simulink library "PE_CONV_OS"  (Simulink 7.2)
settings: Solver=ode45  SolverMode=SingleTasking  StartTime=0.0  StopTime=10.0  RelTol=1e-3
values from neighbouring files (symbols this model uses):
  C = 10e-3*1    (= 0.01)    [INIT_B6_2L_3Ph_IGBT_OS.m]    (also in INIT_B6_3L_3Ph_IGBT_OS.m; INIT_MMC_100L.m = 0.005; INIT_MMC_200L.m = 0.005; INIT_MMC_20L.m)
  FS = 900    [INIT_B6_2L_3Ph_IGBT_OS.m]    (also in INIT_B6_3L_3Ph_IGBT_OS.m; INIT_PWM_2L.m = 1000; INIT_PWM_3L.m = 1000; INIT_PWM_Con.m = 1000)
  LN = 2e-3    (= 0.002)    [INIT_PWM_2L.m]    (also in INIT_PWM_3L.m; INIT_PWM_Con.m; INIT_MMC_100L.m = 0.025; INIT_MMC_200L.m = 0.025)
  LS = 1e-3    (= 0.001)    [INIT_B6_2L_3Ph_IGBT_OS.m]    (also in INIT_B6_3L_3Ph_IGBT_OS.m; INIT_MMC_100L.m = 0.025; INIT_MMC_200L.m = 0.025; INIT_MMC_20L.m = 0.0025)
  LT = LN    (= 0.025)    [INIT_MMC_100L.m]    (also in INIT_MMC_200L.m; INIT_MMC_20L.m = 0.002; INIT_MMC_400L.m)
  Nc = 100    [INIT_MMC_100L.m]    (also in INIT_MMC_200L.m = 200; INIT_MMC_20L.m = 20; INIT_MMC_400L.m = 400)
  NT = sqrt(3)*340/400    [INIT_MMC_100L.m]    (also in INIT_MMC_200L.m; INIT_MMC_20L.m = sqrt(3); INIT_MMC_400L.m)
  Rg = 1e-3    (= 0.001)    [INIT_MMC_100L.m]    (also in INIT_MMC_200L.m; INIT_MMC_20L.m; INIT_MMC_400L.m)
  RN = 0.1    [INIT_PWM_2L.m]    (also in INIT_PWM_3L.m; INIT_PWM_Con.m; INIT_MMC_100L.m; INIT_MMC_200L.m)
  RT = RN    (= 0.1)    [INIT_MMC_100L.m]    (also in INIT_MMC_200L.m; INIT_MMC_20L.m; INIT_MMC_400L.m)
  UC0 = 600    [INIT_B6_2L_3Ph_IGBT_OS.m]    (also in INIT_B6_3L_3Ph_IGBT_OS.m = 500; INIT_MMC_100L.m = 6800; INIT_MMC_200L.m = 3400; INIT_MMC_20L.m = 5000)
undefined symbols (not defined in the file or in its folder): A, DT, FT, L, O1, O2, PHT, T, Td
libraries: simulink_extras x2
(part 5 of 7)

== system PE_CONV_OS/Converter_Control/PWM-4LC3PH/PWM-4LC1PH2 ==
  In1 : Inport  OutDataType=sfix(16)  OutScaling=2^0
  Mux : Mux  Inputs=6
  PWM-2L-1PH : Subsystem  mask(PWM-2L-1PH){FT=FT, PHT=PHT1, DT=DT}
      mask prompts: FT "Triangular Frequency"; PHT "Trian. Phase Angle (Degree)"; DT "Dead Time"
      mask help: Pulse Width Modulation for 1 Phase Converter
  PWM-2L-1PH1 : Subsystem  mask(PWM-2L-1PH){FT=FT, PHT=PHT2, DT=DT}
      mask prompts: FT "Triangular Frequency"; PHT "Trian. Phase Angle (Degree)"; DT "Dead Time"
      mask help: Pulse Width Modulation for 1 Phase Converter
  PWM-2L-1PH2 : Subsystem  mask(PWM-2L-1PH){FT=FT, PHT=PHT3, DT=DT}
      mask prompts: FT "Triangular Frequency"; PHT "Trian. Phase Angle (Degree)"; DT "Dead Time"
      mask help: Pulse Width Modulation for 1 Phase Converter
  Out1 : Outport
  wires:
  PWM-2L-1PH/2(Out2) -> Mux/6
  In1/1 -> PWM-2L-1PH/1(In1), PWM-2L-1PH1/1(In1), PWM-2L-1PH2/1(In1)
  Mux/1 -> Out1/1
  PWM-2L-1PH2/2(Out2) -> Mux/4
  PWM-2L-1PH2/1(Out1) -> Mux/3
  PWM-2L-1PH1/2(Out2) -> Mux/5
  PWM-2L-1PH1/1(Out1) -> Mux/2
  PWM-2L-1PH/1(Out1) -> Mux/1

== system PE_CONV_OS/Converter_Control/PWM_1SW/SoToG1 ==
  Clock : Clock
  P : Product  OutDataType=sfix(16)  OutScaling=2^0
  T1 : Constant  Value=T  OutDataType=sfix(16)  OutScaling=2^0
  T2 : Constant  Value=1/T  OutDataType=sfix(16)  OutScaling=2^0
  mod : Math  Operator=mod
  O : Outport
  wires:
  P/1 -> O/1
  mod/1 -> P/1
  T2/1 -> P/2
  T1/1 -> mod/2
  Clock/1 -> mod/1

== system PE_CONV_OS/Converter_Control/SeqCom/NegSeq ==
  In1 : Inport  OutDataType=sfix(16)  OutScaling=2^0
  Demux : Demux  Outputs=3
  Gain : Gain  Gain=1/3  ParameterDataType=sfix(16)  ParameterScaling=2^0  OutDataType=sfix(16)  OutScaling=2^0
  Gain1 : Gain  Gain=1/3  ParameterDataType=sfix(16)  ParameterScaling=2^0  OutDataType=sfix(16)  OutScaling=2^0
  Gain2 : Gain  Gain=1/3  ParameterDataType=sfix(16)  ParameterScaling=2^0  OutDataType=sfix(16)  OutScaling=2^0
  Mux : Mux  Inputs=3
  Sum : Sum  Inputs=+++  OutDataType=sfix(16)  OutScaling=2^0
  Sum1 : Sum  Inputs=+++  OutDataType=sfix(16)  OutScaling=2^0
  Sum2 : Sum  Inputs=+++  OutDataType=sfix(16)  OutScaling=2^0
  TD : TransportDelay  DelayTime=T/3  BufferSize=BF
  TD1 : TransportDelay  DelayTime=2*T/3  BufferSize=BF
  TD2 : TransportDelay  DelayTime=2*T/3  BufferSize=BF
  TD3 : TransportDelay  DelayTime=T/3  BufferSize=BF
  TD4 : TransportDelay  DelayTime=T/3  BufferSize=BF
  TD5 : TransportDelay  DelayTime=2*T/3  BufferSize=BF
  Out1 : Outport
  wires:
  Gain2/1 -> Mux/3
  Gain1/1 -> Mux/2
  Sum/1 -> Gain/1
  Demux/1 -> Sum/1, TD2/1, TD4/1
  TD1/1 -> Sum/3
  TD/1 -> Sum/2
  Demux/3 -> TD1/1, TD3/1, Sum2/3
  Demux/2 -> TD/1, Sum1/2, TD5/1
  In1/1 -> Demux/1
  TD2/1 -> Sum1/1
  TD3/1 -> Sum1/3
  Sum1/1 -> Gain1/1
  Gain/1 -> Mux/1
  Mux/1 -> Out1/1
  Sum2/1 -> Gain2/1
  TD4/1 -> Sum2/1
  TD5/1 -> Sum2/2

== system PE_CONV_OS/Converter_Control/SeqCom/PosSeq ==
  In1 : Inport  OutDataType=sfix(16)  OutScaling=2^0
  Demux : Demux  Outputs=3
  Gain : Gain  Gain=1/3  ParameterDataType=sfix(16)  ParameterScaling=2^0  OutDataType=sfix(16)  OutScaling=2^0
  Gain1 : Gain  Gain=1/3  ParameterDataType=sfix(16)  ParameterScaling=2^0  OutDataType=sfix(16)  OutScaling=2^0
  Gain2 : Gain  Gain=1/3  ParameterDataType=sfix(16)  ParameterScaling=2^0  OutDataType=sfix(16)  OutScaling=2^0
  Mux : Mux  Inputs=3
  Sum : Sum  Inputs=+++  OutDataType=sfix(16)  OutScaling=2^0
  Sum1 : Sum  Inputs=+++  OutDataType=sfix(16)  OutScaling=2^0
  Sum2 : Sum  Inputs=+++  OutDataType=sfix(16)  OutScaling=2^0
  TD : TransportDelay  DelayTime=2*T/3  BufferSize=BF
  TD1 : TransportDelay  DelayTime=T/3  BufferSize=BF
  TD2 : TransportDelay  DelayTime=T/3  BufferSize=BF
  TD3 : TransportDelay  DelayTime=2*T/3  BufferSize=BF
  TD4 : TransportDelay  DelayTime=2*T/3  BufferSize=BF
  TD5 : TransportDelay  DelayTime=T/3  BufferSize=BF
  Out1 : Outport
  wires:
  Gain2/1 -> Mux/3
  TD5/1 -> Sum2/2
  TD4/1 -> Sum2/1
  Sum2/1 -> Gain2/1
  Mux/1 -> Out1/1
  Gain1/1 -> Mux/2
  Gain/1 -> Mux/1
  Sum1/1 -> Gain1/1
  TD3/1 -> Sum1/3
  TD2/1 -> Sum1/1
  In1/1 -> Demux/1
  Demux/2 -> TD5/1, Sum1/2, TD/1
  Demux/3 -> Sum2/3, TD3/1, TD1/1
  TD/1 -> Sum/2
  TD1/1 -> Sum/3
  Demux/1 -> TD4/1, TD2/1, Sum/1
  Sum/1 -> Gain/1

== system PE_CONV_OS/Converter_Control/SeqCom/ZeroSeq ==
  In1 : Inport  OutDataType=sfix(16)  OutScaling=2^0
  Demux : Demux  Outputs=3
  Gain : Gain  Gain=1/3  ParameterDataType=sfix(16)  ParameterScaling=2^0  OutDataType=sfix(16)  OutScaling=2^0
  Mux : Mux  Inputs=3
  Sum : Sum  Inputs=+++  OutDataType=sfix(16)  OutScaling=2^0
  Out1 : Outport
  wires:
  Mux/1 -> Out1/1
  Gain/1 -> Mux/3, Mux/1, Mux/2
  In1/1 -> Demux/1
  Sum/1 -> Gain/1
  Demux/1 -> Sum/1
  Demux/2 -> Sum/2
  Demux/3 -> Sum/3

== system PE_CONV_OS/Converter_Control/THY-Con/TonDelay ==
  s1 : Inport  Orientation=down  OutDataType=sfix(16)  OutScaling=2^0
  Int : Integrator  ExternalReset=falling
  Rel1 : Relay  OnSwitchValue=DT  OutDataType=sfix(16)  OutScaling=2^0
  s1d : Outport  InitialOutput=0
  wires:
  Rel1/1 -> s1d/1
  s1/1 -> Int/1, Int/2
  Int/1 -> Rel1/1

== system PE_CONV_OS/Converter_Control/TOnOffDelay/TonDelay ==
  s1 : Inport  Orientation=down  OutDataType=sfix(16)  OutScaling=2^0
  Int : Integrator  ExternalReset=falling
  Rel1 : Relay  OnSwitchValue=DT  OutDataType=sfix(16)  OutScaling=2^0
  s1d : Outport  InitialOutput=0
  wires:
  Rel1/1 -> s1d/1
  s1/1 -> Int/1, Int/2
  Int/1 -> Rel1/1

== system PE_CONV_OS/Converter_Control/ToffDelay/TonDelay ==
  s1 : Inport  Orientation=down  OutDataType=sfix(16)  OutScaling=2^0
  Int : Integrator  ExternalReset=falling
  Rel1 : Relay  OnSwitchValue=DT  OutDataType=sfix(16)  OutScaling=2^0
  s1d : Outport  InitialOutput=0
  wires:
  Int/1 -> Rel1/1
  s1/1 -> Int/2, Int/1
  Rel1/1 -> s1d/1

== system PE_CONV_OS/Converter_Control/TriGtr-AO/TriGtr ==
  Clock : Clock
  S1 : Subsystem
  Sum : Sum
  T : Constant  Value=T
  Td : Constant  Value=Td
  mod : Math  Operator=mod
  O : Outport  InitialOutput=0
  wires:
  mod/1 -> S1/1(I1)
  S1/1(O1) -> O/1
  Clock/1 -> Sum/1
  T/1 -> mod/2
  Sum/1 -> mod/1
  Td/1 -> Sum/2

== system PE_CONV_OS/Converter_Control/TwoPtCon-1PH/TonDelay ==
  s1 : Inport  Orientation=down  OutDataType=sfix(16)  OutScaling=2^0
  Int : Integrator  ExternalReset=falling
  Rel1 : Relay  OnSwitchValue=DT  OutDataType=sfix(16)  OutScaling=2^0
  s1d : Outport  InitialOutput=0
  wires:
  Rel1/1 -> s1d/1
  s1/1 -> Int/1, Int/2
  Int/1 -> Rel1/1

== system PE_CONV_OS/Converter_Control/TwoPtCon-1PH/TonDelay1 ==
  s1 : Inport  Orientation=down  OutDataType=sfix(16)  OutScaling=2^0
  Int : Integrator  ExternalReset=falling
  Rel1 : Relay  OnSwitchValue=DT  OutDataType=sfix(16)  OutScaling=2^0
  s1d : Outport  InitialOutput=0
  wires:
  Rel1/1 -> s1d/1
  s1/1 -> Int/1, Int/2
  Int/1 -> Rel1/1

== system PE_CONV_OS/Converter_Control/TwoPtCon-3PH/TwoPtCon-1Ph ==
  In1 : Inport  OutDataType=sfix(16)  OutScaling=2^0
  In2 : Inport  Port=2  OutDataType=sfix(16)  OutScaling=2^0
  DT : DataTypeConversion
  DT1 : DataTypeConversion
  Relay : Relay  OnSwitchValue=SP  OffSwitchValue=SN  OutDataType=sfix(16)  OutScaling=2^0
  Sum : Sum  Inputs=+-  OutDataType=sfix(16)  OutScaling=2^0
  TonDelay : Subsystem  mask(TonDelay){DT=DT}
      mask prompts: DT "Dead Time"
      mask help: Turn on dead time to protect against short circuit of the converter leg
  TonDelay1 : Subsystem  mask(TonDelay){DT=DT}
      mask prompts: DT "Dead Time"
      mask help: Turn on dead time to protect against short circuit of the converter leg
  not : Logic  Operator=NOT  Inputs=1
  Out1 : Outport  InitialOutput=0
  Out2 : Outport  Port=2  InitialOutput=0
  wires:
  In1/1 -> Sum/1
  In2/1 -> Sum/2
  Sum/1 -> Relay/1
  not/1 -> DT/1
  Relay/1 -> TonDelay/1(s1), DT1/1
  TonDelay1/1(s1d) -> Out2/1
  TonDelay/1(s1d) -> Out1/1
  DT/1 -> TonDelay1/1(s1)
  DT1/1 -> not/1

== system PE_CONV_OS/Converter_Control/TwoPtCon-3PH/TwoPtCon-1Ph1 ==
  In1 : Inport  OutDataType=sfix(16)  OutScaling=2^0
  In2 : Inport  Port=2  OutDataType=sfix(16)  OutScaling=2^0
  DT : DataTypeConversion
  DT1 : DataTypeConversion
  Relay : Relay  OnSwitchValue=SP  OffSwitchValue=SN  OutDataType=sfix(16)  OutScaling=2^0
  Sum : Sum  Inputs=+-  OutDataType=sfix(16)  OutScaling=2^0
  TonDelay : Subsystem  mask(TonDelay){DT=DT}
      mask prompts: DT "Dead Time"
      mask help: Turn on dead time to protect against short circuit of the converter leg
  TonDelay1 : Subsystem  mask(TonDelay){DT=DT}
      mask prompts: DT "Dead Time"
      mask help: Turn on dead time to protect against short circuit of the converter leg
  not : Logic  Operator=NOT  Inputs=1
  Out1 : Outport  InitialOutput=0
  Out2 : Outport  Port=2  InitialOutput=0
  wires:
  In1/1 -> Sum/1
  In2/1 -> Sum/2
  Sum/1 -> Relay/1
  not/1 -> DT/1
  Relay/1 -> TonDelay/1(s1), DT1/1
  TonDelay1/1(s1d) -> Out2/1
  TonDelay/1(s1d) -> Out1/1
  DT/1 -> TonDelay1/1(s1)
  DT1/1 -> not/1

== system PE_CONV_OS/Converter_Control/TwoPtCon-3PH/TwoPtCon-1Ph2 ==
  In1 : Inport  OutDataType=sfix(16)  OutScaling=2^0
  In2 : Inport  Port=2  OutDataType=sfix(16)  OutScaling=2^0
  DT : DataTypeConversion
  DT1 : DataTypeConversion
  Relay : Relay  OnSwitchValue=SP  OffSwitchValue=SN  OutDataType=sfix(16)  OutScaling=2^0
  Sum : Sum  Inputs=+-  OutDataType=sfix(16)  OutScaling=2^0
  TonDelay : Subsystem  mask(TonDelay){DT=DT}
      mask prompts: DT "Dead Time"
      mask help: Turn on dead time to protect against short circuit of the converter leg
  TonDelay1 : Subsystem  mask(TonDelay){DT=DT}
      mask prompts: DT "Dead Time"
      mask help: Turn on dead time to protect against short circuit of the converter leg
  not : Logic  Operator=NOT  Inputs=1
  Out1 : Outport  InitialOutput=0
  Out2 : Outport  Port=2  InitialOutput=0
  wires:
  In1/1 -> Sum/1
  In2/1 -> Sum/2
  Sum/1 -> Relay/1
  not/1 -> DT/1
  Relay/1 -> TonDelay/1(s1), DT1/1
  TonDelay1/1(s1d) -> Out2/1
  TonDelay/1(s1d) -> Out1/1
  DT/1 -> TonDelay1/1(s1)
  DT1/1 -> not/1

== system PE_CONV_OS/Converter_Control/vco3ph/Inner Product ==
  in_1 : Inport  OutDataType=sfix(16)  OutScaling=2^0
  in_2 : Inport  Port=2  OutDataType=sfix(16)  OutScaling=2^0
  Product : Product  OutDataType=sfix(16)  OutScaling=2^0
  Sum : Sum  Inputs=+  OutDataType=sfix(16)  OutScaling=2^0
  out_1 : Outport  InitialOutput=0
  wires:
  Sum/1 -> out_1/1
  Product/1 -> Sum/1
  in_1/1 -> Product/1
  in_2/1 -> Product/2

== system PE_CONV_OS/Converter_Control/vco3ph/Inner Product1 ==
  in_1 : Inport  OutDataType=sfix(16)  OutScaling=2^0
  in_2 : Inport  Port=2  OutDataType=sfix(16)  OutScaling=2^0
  Product : Product  OutDataType=sfix(16)  OutScaling=2^0
  Sum : Sum  Inputs=+  OutDataType=sfix(16)  OutScaling=2^0
  out_1 : Outport  InitialOutput=0
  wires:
  Sum/1 -> out_1/1
  Product/1 -> Sum/1
  in_1/1 -> Product/1
  in_2/1 -> Product/2

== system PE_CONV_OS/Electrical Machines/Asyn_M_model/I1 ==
  Phir* : Inport
  KF : Gain  Gain=1/LM
  Id* : Outport
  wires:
  Phir*/1 -> KF/1
  KF/1 -> Id*/1

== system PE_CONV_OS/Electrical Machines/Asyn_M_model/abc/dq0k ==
  abc : Inport
  th : Inport  Port=2
  Demux : Demux  Outputs=3
  Fcn : Fcn  Expr=u(1)*cos(u(3)) + u(2)*sin(u(3))
  Fcn1 : Fcn  Expr=-u(1)*sin(u(3)) + u(2)*cos(u(3))
  K : Gain  Gain="2/3*[1   -.5   -.5;  0   sqrt(3)/2   -sqrt(3)/2;  .5    .5    .5]"  Multiplication=Matrix(K*u)
  Mux1 : Mux  Inputs=3
  dk : Outport
  qk : Outport  Port=2
  0k : Outport  Port=3
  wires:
  abc/1 -> K/1
  Demux/2 -> Mux1/2
  Demux/1 -> Mux1/1
  Demux/3 -> 0k/1
  th/1 -> Mux1/3
  Fcn1/1 -> qk/1
  Fcn/1 -> dk/1
  Mux1/1 -> Fcn/1, Fcn1/1
  K/1 -> Demux/1

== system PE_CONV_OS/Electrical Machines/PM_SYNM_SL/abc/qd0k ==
  a : Inport  OutDataType=sfix(16)  OutScaling=2^0
  b : Inport  Port=2  OutDataType=sfix(16)  OutScaling=2^0
  c : Inport  Port=3  OutDataType=sfix(16)  OutScaling=2^0
  th : Inport  Port=4  OutDataType=sfix(16)  OutScaling=2^0
  Demux : Demux  Outputs=3
  Fcn : Fcn  Expr=u(1)*cos(u(3)) - u(2)*sin(u(3))
  Fcn1 : Fcn  Expr=u(1)*sin(u(3)) + u(2)*cos(u(3))
  K : Gain  Gain="2/3*[1   -.5   -.5;  0   -sqrt(3)/2   sqrt(3)/2;  .5    .5    .5]"  Multiplication=Matrix(K*u)  ParameterDataType=sfix(16)  ParameterScaling=2^0  OutDataType=sfix(16)  OutScaling=2^0
  Mux : Mux  Inputs=3
  Mux1 : Mux  Inputs=3
  qk : Outport
  dk : Outport  Port=2
  0k : Outport  Port=3
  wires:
  Demux/2 -> Mux1/2
  Demux/1 -> Mux1/1
  Demux/3 -> 0k/1
  th/1 -> Mux1/3
  Fcn1/1 -> dk/1
  Fcn/1 -> qk/1
  Mux1/1 -> Fcn/1, Fcn1/1
  a/1 -> Mux/1
  Mux/1 -> K/1
  K/1 -> Demux/1
  b/1 -> Mux/2
  c/1 -> Mux/3

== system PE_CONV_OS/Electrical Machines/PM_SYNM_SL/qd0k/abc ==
  qk : Inport  OutDataType=sfix(16)  OutScaling=2^0
  dk : Inport  Port=2  OutDataType=sfix(16)  OutScaling=2^0
  0k : Inport  Port=3  OutDataType=sfix(16)  OutScaling=2^0
  th : Inport  Port=4  OutDataType=sfix(16)  OutScaling=2^0
  Demux : Demux  Outputs=3
  Fcn : Fcn  Expr=u(1)*cos(u(3)) + u(2)*sin(u(3))
  Fcn1 : Fcn  Expr=-u(1)*sin(u(3)) + u(2)*cos(u(3))
  K : Gain  Gain="[1   0  1 ;  -.5   -sqrt(3)/2    1 ;  -.5    sqrt(3)/2    1]"  Multiplication=Matrix(K*u)  ParameterDataType=sfix(16)  ParameterScaling=2^0  OutDataType=sfix(16)  OutScaling=2^0
  Mux : Mux  Inputs=3
  Mux1 : Mux  Inputs=3
  a : Outport
  b : Outport  Port=2
  c : Outport  Port=3
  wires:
  0k/1 -> Mux1/3
  th/1 -> Mux/3
  Demux/3 -> c/1
  Demux/2 -> b/1
  Demux/1 -> a/1
  Fcn1/1 -> Mux1/2
  Fcn/1 -> Mux1/1
  Mux1/1 -> K/1
  K/1 -> Demux/1
  Mux/1 -> Fcn1/1, Fcn/1
  dk/1 -> Mux/2
  qk/1 -> Mux/1

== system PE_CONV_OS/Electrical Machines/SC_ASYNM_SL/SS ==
  note: psiqs
  note: psiqm
  note: psiqr
  note: iqr
  note: iqs
  uqs : Inport
  wr*psidr : Inport  Port=2
  F : Fcn  Expr=u(1)-rs*u(2)
  F1 : Fcn  Expr=u(1)-rr*u(2)+u(3)
  F2 : Fcn  Expr=u(3)*((u(1)/Lls)+(u(2)/Llr))
  F3 : Fcn  Expr=(1/Lls)*(u(1)-u(2))
  F4 : Fcn  Expr=-(1/Llr)*(u(1)-u(2))
  F5 : Fcn  Expr=u(1)
  F6 : Fcn  Expr=u(2)
  I : Integrator
  I1 : Integrator
  LM : Constant  Value=1/(1/Lls+ 1/Llr+ 1/Lm)
  Mux : Mux  Inputs=2
  Mux1 : Mux  Inputs=3
  Mux2 : Mux  Inputs=3
  Mux3 : Mux  Inputs=2
  Mux4 : Mux  Inputs=2
  uqr : Constant  Value=0
  psiqs : Outport
  iqs : Outport  Port=2
  psiqr : Outport  Port=3
  iqr : Outport  Port=4
  psiqm : Outport  Port=5
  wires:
  Mux/1 -> F/1
  F/1 -> I/1
  Mux1/1 -> F1/1
  Mux2/1 -> F2/1
  F2/1 -> Mux3/2, Mux4/1, psiqm/1
  I/1 -> Mux2/1, Mux3/1
  I1/1 -> Mux4/2, Mux2/2
  uqs/1 -> Mux/1
  Mux3/1 -> F3/1, F5/1
  F5/1 -> psiqs/1
  Mux4/1 -> F4/1, F6/1
  F6/1 -> psiqr/1
  F1/1 -> I1/1
  uqr/1 -> Mux1/1
  F3/1 -> iqs/1, Mux/2
  wr*psidr/1 -> Mux1/3
  F4/1 -> iqr/1, Mux1/2
  LM/1 -> Mux2/3

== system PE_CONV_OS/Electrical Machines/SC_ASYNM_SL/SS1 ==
  note: ids
  note: idr
  uds : Inport
  wr*psiqr : Inport  Port=2
  F : Fcn  Expr=u(1)-rs*u(2)
  F1 : Fcn  Expr=u(1)-rr*u(2)-u(3)
  F3 : Fcn  Expr=(1/Lls)*(u(1)-u(2))
  F4 : Fcn  Expr=-(1/Llr)*(u(1)-u(2))
  F5 : Fcn  Expr=u(1)
  F6 : Fcn  Expr=u(2)
  I : Integrator
  I1 : Integrator
  LM : Constant  Value=1/(1/Lls+ 1/Llr+ 1/Lm)
  Mux : Mux  Inputs=2
  Mux1 : Mux  Inputs=3
  Mux2 : Mux  Inputs=3
  Mux3 : Mux  Inputs=2
  Mux4 : Mux  Inputs=2
  psidm2 : Fcn  Expr=u(3)*(u(1)/Lls+u(2)/Llr)
  udr : Constant  Value=0
  psids : Outport
  ids : Outport  Port=2
  psidr : Outport  Port=3
  idr : Outport  Port=4
  psidm : Outport  Port=5
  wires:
  F6/1 -> psidr/1
  Mux4/1 -> F6/1, F4/1
  F5/1 -> psids/1
  Mux3/1 -> F5/1, F3/1
  uds/1 -> Mux/1
  I1/1 -> Mux4/2, Mux2/2
  I/1 -> Mux3/1, Mux2/1
  Mux2/1 -> psidm2/1
  Mux1/1 -> F1/1
  F/1 -> I/1
  Mux/1 -> F/1
  F1/1 -> I1/1
  wr*psiqr/1 -> Mux1/3
  udr/1 -> Mux1/1
  F3/1 -> ids/1, Mux/2
  F4/1 -> idr/1, Mux1/2
  LM/1 -> Mux2/3
  psidm2/1 -> Mux3/2, Mux4/1, psidm/1

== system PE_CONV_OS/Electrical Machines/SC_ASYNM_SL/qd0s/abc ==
  q : Inport
  d : Inport  Port=2
  0 : Inport  Port=3
  Demux : Demux  Outputs=3
  K : Gain  Gain="[1   0  1;  -.5   -sqrt(3)/2   1;  -.5    sqrt(3)/2  1]"  Multiplication=Matrix(K*u)
  Mux : Mux  Inputs=3
  a : Outport
  b : Outport  Port=2
  c : Outport  Port=3
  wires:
  Demux/1 -> a/1
  q/1 -> Mux/1
  0/1 -> Mux/3
  Demux/3 -> c/1
  Demux/2 -> b/1
  Mux/1 -> K/1
  K/1 -> Demux/1
  d/1 -> Mux/2

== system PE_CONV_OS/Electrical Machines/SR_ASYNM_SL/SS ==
  note: iqs
  note: iqr
  note: psiqr
  note: psiqm
  note: psiqs
  uqs : Inport
  uqr : Inport  Port=2
  wr*ps : Inport  Port=3
  F : Fcn  Expr=u(1)-rs*u(2)
  F1 : Fcn  Expr=u(1)-rr*u(2)+u(3)
  F2 : Fcn  Expr=u(3)*((u(1)/Lls)+(u(2)/Llr))
  F3 : Fcn  Expr=(1/Lls)*(u(1)-u(2))
  F4 : Fcn  Expr=-(1/Llr)*(u(1)-u(2))
  F5 : Fcn  Expr=u(1)
  F6 : Fcn  Expr=u(2)
  I : Integrator
  I1 : Integrator
  LM : Constant  Value=1/(1/Lls+ 1/Llr+ 1/Lm)
  Mux : Mux  Inputs=2
  Mux1 : Mux  Inputs=3
  Mux2 : Mux  Inputs=3
  Mux3 : Mux  Inputs=2
  Mux4 : Mux  Inputs=2
  psiqs : Outport
  iqs : Outport  Port=2
  psiqr : Outport  Port=3
  iqr : Outport  Port=4
  psiqm : Outport  Port=5
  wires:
  LM/1 -> Mux2/3
  F4/1 -> Mux1/2, iqr/1
  wr*ps/1 -> Mux1/3
  F3/1 -> Mux/2, iqs/1
  uqr/1 -> Mux1/1
  F1/1 -> I1/1
  F6/1 -> psiqr/1
  Mux4/1 -> F6/1, F4/1
  F5/1 -> psiqs/1
  Mux3/1 -> F5/1, F3/1
  uqs/1 -> Mux/1
  I1/1 -> Mux2/2, Mux4/2
  I/1 -> Mux3/1, Mux2/1
  F2/1 -> psiqm/1, Mux4/1, Mux3/2
  Mux2/1 -> F2/1
  Mux1/1 -> F1/1
  F/1 -> I/1
  Mux/1 -> F/1

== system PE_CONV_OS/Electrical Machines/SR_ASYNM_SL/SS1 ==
  note: idr
  note: ids
  uds : Inport
  udr : Inport  Port=2
  wr*ps : Inport  Port=3
  F : Fcn  Expr=u(1)-rs*u(2)
  F1 : Fcn  Expr=u(1)-rr*u(2)-u(3)
  F3 : Fcn  Expr=(1/Lls)*(u(1)-u(2))
  F4 : Fcn  Expr=-(1/Llr)*(u(1)-u(2))
  F5 : Fcn  Expr=u(1)
  F6 : Fcn  Expr=u(2)
  I : Integrator
  I1 : Integrator
  LM : Constant  Value=1/(1/Lls+ 1/Llr+ 1/Lm)
  Mux : Mux  Inputs=2
  Mux1 : Mux  Inputs=3
  Mux2 : Mux  Inputs=3
  Mux3 : Mux  Inputs=2
  Mux4 : Mux  Inputs=2
  psidm2 : Fcn  Expr=u(3)*(u(1)/Lls+u(2)/Llr)
  psids : Outport
  ids : Outport  Port=2
  psidr : Outport  Port=3
  idr : Outport  Port=4
  psidm : Outport  Port=5
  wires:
  psidm2/1 -> psidm/1, Mux4/1, Mux3/2
  LM/1 -> Mux2/3
  F4/1 -> Mux1/2, idr/1
  F3/1 -> Mux/2, ids/1
  udr/1 -> Mux1/1
  wr*ps/1 -> Mux1/3
  F1/1 -> I1/1
  Mux/1 -> F/1
  F/1 -> I/1
  Mux1/1 -> F1/1
  Mux2/1 -> psidm2/1
  I/1 -> Mux2/1, Mux3/1
  I1/1 -> Mux2/2, Mux4/2
  uds/1 -> Mux/1
  Mux3/1 -> F3/1, F5/1
  F5/1 -> psids/1
  Mux4/1 -> F4/1, F6/1
  F6/1 -> psidr/1

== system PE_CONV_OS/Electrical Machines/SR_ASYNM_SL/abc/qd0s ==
  a : Inport
  Demux : Demux  Outputs=3
  K : Gain  Gain="2/3*[1   -.5   -.5;  0   -sqrt(3)/2   sqrt(3)/2;  .5    .5    .5]"  Multiplication=Matrix(K*u)
  q : Outport
  d : Outport  Port=2
  0 : Outport  Port=3
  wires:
  Demux/3 -> 0/1
  Demux/2 -> d/1
  Demux/1 -> q/1
  a/1 -> K/1
  K/1 -> Demux/1

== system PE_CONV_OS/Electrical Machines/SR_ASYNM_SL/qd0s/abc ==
  q : Inport
  d : Inport  Port=2
  0 : Inport  Port=3
  K : Gain  Gain="[1   0  1;  -.5   -sqrt(3)/2   1;  -.5    sqrt(3)/2  1]"  Multiplication=Matrix(K*u)
  Mux : Mux  Inputs=3
  a : Outport
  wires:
  d/1 -> Mux/2
  K/1 -> a/1
  Mux/1 -> K/1
  0/1 -> Mux/3
  q/1 -> Mux/1

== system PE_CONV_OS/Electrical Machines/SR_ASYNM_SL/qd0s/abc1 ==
  q : Inport
  d : Inport  Port=2
  0 : Inport  Port=3
  K : Gain  Gain="[1   0  1;  -.5   -sqrt(3)/2   1;  -.5    sqrt(3)/2  1]"  Multiplication=Matrix(K*u)
  Mux : Mux  Inputs=3
  a : Outport
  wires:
  q/1 -> Mux/1
  0/1 -> Mux/3
  Mux/1 -> K/1
  K/1 -> a/1
  d/1 -> Mux/2

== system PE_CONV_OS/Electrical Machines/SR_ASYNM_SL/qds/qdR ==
  qs : Inport  OutDataType=sfix(16)  OutScaling=2^0
  ds : Inport  Port=2  OutDataType=sfix(16)  OutScaling=2^0
  0s : Inport  Port=3  OutDataType=sfix(16)  OutScaling=2^0
  th : Inport  Port=4  OutDataType=sfix(16)  OutScaling=2^0
  Fcn : Fcn  Expr=u(1)*cos(u(3)) - u(2)*sin(u(3))
  Fcn1 : Fcn  Expr=u(1)*sin(u(3)) + u(2)*cos(u(3))
  Mux : Mux  Inputs=3
  qk : Outport
  dk : Outport  Port=2
  0k : Outport  Port=3
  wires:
  th/1 -> Mux/3
  0s/1 -> 0k/1
  qs/1 -> Mux/1
  ds/1 -> Mux/2
  Mux/1 -> Fcn/1, Fcn1/1
  Fcn/1 -> qk/1
  Fcn1/1 -> dk/1

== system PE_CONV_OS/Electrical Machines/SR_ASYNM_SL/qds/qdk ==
  qs : Inport  OutDataType=sfix(16)  OutScaling=2^0
  ds : Inport  Port=2  OutDataType=sfix(16)  OutScaling=2^0
  0s : Inport  Port=3  OutDataType=sfix(16)  OutScaling=2^0
  th : Inport  Port=4  OutDataType=sfix(16)  OutScaling=2^0
  Fcn : Fcn  Expr=u(1)*cos(u(3)) - u(2)*sin(u(3))
  Fcn1 : Fcn  Expr=u(1)*sin(u(3)) + u(2)*cos(u(3))
  Mux : Mux  Inputs=3
  qk : Outport
  dk : Outport  Port=2
  0k : Outport  Port=3
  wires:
  th/1 -> Mux/3
  0s/1 -> 0k/1
  qs/1 -> Mux/1
  ds/1 -> Mux/2
  Mux/1 -> Fcn/1, Fcn1/1
  Fcn/1 -> qk/1
  Fcn1/1 -> dk/1

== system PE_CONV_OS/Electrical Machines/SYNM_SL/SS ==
  note: iqs
  note: ikq
  note: psiqk
  note: psiqs
  uqs : Inport
  wr*psids : Inport  Port=2
  F : Fcn  Expr=u(1)-rs*u(2)-u(3)
  F1 : Fcn  Expr=u(1)-rk*u(2)
  F2 : Fcn  Expr=u(3)*((u(1)/Lls)+(u(2)/Llkq))
  F3 : Fcn  Expr=(1/Lls)*(u(1)-u(2))
  F4 : Fcn  Expr=(1/Llkq)*(u(2)-u(1))
  F5 : Fcn  Expr=u(1)
  F6 : Fcn  Expr=u(2)
  I : Integrator
  I1 : Integrator
  LMQ : Constant  Value=1/(1/Lls+ 1/Llkq+ 1/Lmq)
  Mux : Mux  Inputs=3
  Mux1 : Mux  Inputs=2
  Mux2 : Mux  Inputs=3
  Mux3 : Mux  Inputs=2
  Mux4 : Mux  Inputs=2
  ukq : Constant  Value=0
  psiqs : Outport
  iqs : Outport  Port=2
  iqk : Outport  Port=3
  psiqm : Outport  Port=4
  psiqk : Outport  Port=5
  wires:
  LMQ/1 -> Mux2/3
  ukq/1 -> Mux1/1
  F1/1 -> I1/1
  uqs/1 -> Mux/1
  I1/1 -> Mux2/2, Mux4/2
  I/1 -> Mux3/1, Mux2/1
  Mux2/1 -> F2/1
  Mux1/1 -> F1/1
  F/1 -> I/1
  Mux/1 -> F/1
  wr*psids/1 -> Mux/3
  F4/1 -> Mux1/2, iqk/1
  F3/1 -> Mux/2, iqs/1
  Mux4/1 -> F6/1, F4/1
  F5/1 -> psiqs/1
  Mux3/1 -> F5/1, F3/1
  F2/1 -> Mux4/1, Mux3/2, psiqm/1
  F6/1 -> psiqk/1

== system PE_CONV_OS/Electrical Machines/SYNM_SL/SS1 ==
  note: idk
  note: ids
  note: psidk
  note: psids
  note: psidf
  note: idf
  uds : Inport
  wr*psiqs : Inport  Port=2
  udf : Inport  Port=3
  F : Fcn  Expr=u(1)-rs*u(2)+u(3)
  F1 : Fcn  Expr=u(1)-rk*u(2)
  F2 : Fcn  Expr=u(1)-rf*u(2)
  F3 : Fcn  Expr=(1/Lls)*(u(1)-u(2))
  F4 : Fcn  Expr=(1/Llkd)*(u(2)-u(1))
  F5 : Fcn  Expr=u(1)
  F6 : Fcn  Expr=u(2)
  F7 : Fcn  Expr=(1/Llf)*(u(2)-u(1))
  F8 : Fcn  Expr=u(2)
  I : Integrator
  I1 : Integrator
  I2 : Integrator
  LMD : Constant  Value=1/(1/Lls+ 1/Llf+ 1/Llkd+ 1/Lmd)
  Mux : Mux  Inputs=3
  Mux{1,3..6} (5 alike) : Mux  Inputs=2
  Mux2 : Mux
  psidm1 : Fcn  Expr=u(4)*(u(1)/Lls+u(2)/Llkd+u(3)/Llf)
  udk : Constant  Value=0
  psids : Outport
  ids : Outport  Port=2
  psidk : Outport  Port=3
  idk : Outport  Port=4
  psidm : Outport  Port=5
  psidf : Outport  Port=6
  idf : Outport  Port=7
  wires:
  psidm1/1 -> psidm/1, Mux3/2, Mux4/1, Mux6/1
  F4/1 -> Mux1/2, idk/1
  F3/1 -> Mux/2, ids/1
  udk/1 -> Mux1/1
  F1/1 -> I1/1
  Mux/1 -> F/1
  F/1 -> I/1
  Mux1/1 -> F1/1
  Mux2/1 -> psidm1/1
  I/1 -> Mux2/1, Mux3/1
  I1/1 -> Mux2/2, Mux4/2
  uds/1 -> Mux/1
  Mux3/1 -> F3/1, F5/1
  F5/1 -> psids/1
  Mux4/1 -> F4/1, F6/1
  F6/1 -> psidk/1
  wr*psiqs/1 -> Mux/3
  udf/1 -> Mux5/1
  Mux5/1 -> F2/1
  F2/1 -> I2/1
  F7/1 -> idf/1, Mux5/2
  Mux6/1 -> F8/1, F7/1
  F8/1 -> psidf/1
  I2/1 -> Mux6/2, Mux2/3
  LMD/1 -> Mux2/4

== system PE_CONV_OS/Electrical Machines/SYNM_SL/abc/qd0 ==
  abc : Inport
  Demux : Demux  Outputs=3
  K : Gain  Gain="2/3*[1   -.5   -.5;  0   -sqrt(3)/2   sqrt(3)/2;  .5    .5    .5]"  Multiplication=Matrix(K*u)
  q : Outport
  d : Outport  Port=2
  0 : Outport  Port=3
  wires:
  K/1 -> Demux/1
  abc/1 -> K/1
  Demux/1 -> q/1
  Demux/2 -> d/1
  Demux/3 -> 0/1

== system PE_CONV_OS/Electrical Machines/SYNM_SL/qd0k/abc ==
  qk : Inport
  dk : Inport  Port=2
  0k : Inport  Port=3
  th : Inport  Port=4
  Demux : Demux  Outputs=3
  Fcn : Fcn  Expr=u(1)*cos(u(3)) + u(2)*sin(u(3))
  Fcn1 : Fcn  Expr=-u(1)*sin(u(3)) + u(2)*cos(u(3))
  K : Gain  Gain="[1   0  1 ;  -.5   -sqrt(3)/2    1 ;  -.5    sqrt(3)/2    1]"  Multiplication=Matrix(K*u)
  Mux : Mux  Inputs=3
  Mux1 : Mux  Inputs=3
  a : Outport
  b : Outport  Port=2
  c : Outport  Port=3
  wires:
  0k/1 -> Mux1/3
  th/1 -> Mux/3
  Demux/3 -> c/1
  Demux/2 -> b/1
  Demux/1 -> a/1
  Fcn1/1 -> Mux1/2
  Fcn/1 -> Mux1/1
  Mux1/1 -> K/1
  K/1 -> Demux/1
  Mux/1 -> Fcn1/1, Fcn/1
  dk/1 -> Mux/2
  qk/1 -> Mux/1

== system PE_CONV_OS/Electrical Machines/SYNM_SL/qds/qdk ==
  qs : Inport
  ds : Inport  Port=2
  th : Inport  Port=3
  Fcn : Fcn  Expr=u(1)*cos(u(3)) - u(2)*sin(u(3))
  Fcn1 : Fcn  Expr=u(1)*sin(u(3)) + u(2)*cos(u(3))
  Mux : Mux  Inputs=3
  qk : Outport
  dk : Outport  Port=2
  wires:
  qs/1 -> Mux/1
  ds/1 -> Mux/2
  th/1 -> Mux/3
  Mux/1 -> Fcn/1, Fcn1/1
  Fcn/1 -> qk/1
  Fcn1/1 -> dk/1

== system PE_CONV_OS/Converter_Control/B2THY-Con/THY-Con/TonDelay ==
  s1 : Inport  Orientation=down  OutDataType=sfix(16)  OutScaling=2^0
  Int : Integrator  ExternalReset=falling
  Rel1 : Relay  OnSwitchValue=DT  OutDataType=sfix(16)  OutScaling=2^0
  s1d : Outport  InitialOutput=0
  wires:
  Int/1 -> Rel1/1
  s1/1 -> Int/2, Int/1
  Rel1/1 -> s1d/1

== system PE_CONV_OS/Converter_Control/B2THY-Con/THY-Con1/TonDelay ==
  s1 : Inport  Orientation=down  OutDataType=sfix(16)  OutScaling=2^0
  Int : Integrator  ExternalReset=falling
  Rel1 : Relay  OnSwitchValue=DT  OutDataType=sfix(16)  OutScaling=2^0
  s1d : Outport  InitialOutput=0
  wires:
  Int/1 -> Rel1/1
  s1/1 -> Int/2, Int/1
  Rel1/1 -> s1d/1

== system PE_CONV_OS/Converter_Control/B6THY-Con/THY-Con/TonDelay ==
  s1 : Inport  Orientation=down  OutDataType=sfix(16)  OutScaling=2^0
  Int : Integrator  ExternalReset=falling
  Rel1 : Relay  OnSwitchValue=DT  OutDataType=sfix(16)  OutScaling=2^0
  s1d : Outport  InitialOutput=0
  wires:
  Int/1 -> Rel1/1
  s1/1 -> Int/2, Int/1
  Rel1/1 -> s1d/1

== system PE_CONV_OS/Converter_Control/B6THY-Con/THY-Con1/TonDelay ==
  s1 : Inport  Orientation=down  OutDataType=sfix(16)  OutScaling=2^0
  Int : Integrator  ExternalReset=falling
  Rel1 : Relay  OnSwitchValue=DT  OutDataType=sfix(16)  OutScaling=2^0
  s1d : Outport  InitialOutput=0
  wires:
  Int/1 -> Rel1/1
  s1/1 -> Int/2, Int/1
  Rel1/1 -> s1d/1

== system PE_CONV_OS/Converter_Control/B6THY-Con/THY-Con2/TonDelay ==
  s1 : Inport  Orientation=down  OutDataType=sfix(16)  OutScaling=2^0
  Int : Integrator  ExternalReset=falling
  Rel1 : Relay  OnSwitchValue=DT  OutDataType=sfix(16)  OutScaling=2^0
  s1d : Outport  InitialOutput=0
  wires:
  Int/1 -> Rel1/1
  s1/1 -> Int/2, Int/1
  Rel1/1 -> s1d/1

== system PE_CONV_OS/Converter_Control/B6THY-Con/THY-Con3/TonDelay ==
  s1 : Inport  Orientation=down  OutDataType=sfix(16)  OutScaling=2^0
  Int : Integrator  ExternalReset=falling
  Rel1 : Relay  OnSwitchValue=DT  OutDataType=sfix(16)  OutScaling=2^0
  s1d : Outport  InitialOutput=0
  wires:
  Int/1 -> Rel1/1
  s1/1 -> Int/2, Int/1
  Rel1/1 -> s1d/1

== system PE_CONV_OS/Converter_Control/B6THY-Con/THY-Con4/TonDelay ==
  s1 : Inport  Orientation=down  OutDataType=sfix(16)  OutScaling=2^0
  Int : Integrator  ExternalReset=falling
  Rel1 : Relay  OnSwitchValue=DT  OutDataType=sfix(16)  OutScaling=2^0
  s1d : Outport  InitialOutput=0
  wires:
  Int/1 -> Rel1/1
  s1/1 -> Int/2, Int/1
  Rel1/1 -> s1d/1

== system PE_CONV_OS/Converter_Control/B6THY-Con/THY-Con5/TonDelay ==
  s1 : Inport  Orientation=down  OutDataType=sfix(16)  OutScaling=2^0
  Int : Integrator  ExternalReset=falling
  Rel1 : Relay  OnSwitchValue=DT  OutDataType=sfix(16)  OutScaling=2^0
  s1d : Outport  InitialOutput=0
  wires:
  Int/1 -> Rel1/1
  s1/1 -> Int/2, Int/1
  Rel1/1 -> s1d/1

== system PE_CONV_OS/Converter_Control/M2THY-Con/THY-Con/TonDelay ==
  s1 : Inport  Orientation=down  OutDataType=sfix(16)  OutScaling=2^0
  Int : Integrator  ExternalReset=falling
  Rel1 : Relay  OnSwitchValue=DT  OutDataType=sfix(16)  OutScaling=2^0
  s1d : Outport  InitialOutput=0
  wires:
  Rel1/1 -> s1d/1
  s1/1 -> Int/1, Int/2
  Int/1 -> Rel1/1

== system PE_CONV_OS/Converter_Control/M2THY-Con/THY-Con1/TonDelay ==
  s1 : Inport  Orientation=down  OutDataType=sfix(16)  OutScaling=2^0
  Int : Integrator  ExternalReset=falling
  Rel1 : Relay  OnSwitchValue=DT  OutDataType=sfix(16)  OutScaling=2^0
  s1d : Outport  InitialOutput=0
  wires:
  Int/1 -> Rel1/1
  s1/1 -> Int/2, Int/1
  Rel1/1 -> s1d/1

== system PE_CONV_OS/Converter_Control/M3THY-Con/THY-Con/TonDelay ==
  s1 : Inport  Orientation=down  OutDataType=sfix(16)  OutScaling=2^0
  Int : Integrator  ExternalReset=falling
  Rel1 : Relay  OnSwitchValue=DT  OutDataType=sfix(16)  OutScaling=2^0
  s1d : Outport  InitialOutput=0
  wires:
  Int/1 -> Rel1/1
  s1/1 -> Int/2, Int/1
  Rel1/1 -> s1d/1

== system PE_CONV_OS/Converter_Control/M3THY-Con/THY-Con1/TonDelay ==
  s1 : Inport  Orientation=down  OutDataType=sfix(16)  OutScaling=2^0
  Int : Integrator  ExternalReset=falling
  Rel1 : Relay  OnSwitchValue=DT  OutDataType=sfix(16)  OutScaling=2^0
  s1d : Outport  InitialOutput=0
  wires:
  Rel1/1 -> s1d/1
  s1/1 -> Int/1, Int/2
  Int/1 -> Rel1/1

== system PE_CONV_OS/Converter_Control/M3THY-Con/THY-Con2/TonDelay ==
  s1 : Inport  Orientation=down  OutDataType=sfix(16)  OutScaling=2^0
  Int : Integrator  ExternalReset=falling
  Rel1 : Relay  OnSwitchValue=DT  OutDataType=sfix(16)  OutScaling=2^0
  s1d : Outport  InitialOutput=0
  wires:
  Rel1/1 -> s1d/1
  s1/1 -> Int/1, Int/2
  Int/1 -> Rel1/1

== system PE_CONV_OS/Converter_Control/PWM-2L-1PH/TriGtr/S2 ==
  I1 : Inport
  Fcn : Fcn  Expr="(u* (u <=T/4) * 4/T)   +  (  (u > T/4) && ( u <=3*T/4) )* ( 1 - (u-T/4) *4/T )   +  ( (u > 3*T/4)&& (u<=T)) * ( ((u -3*T/4)* 4/T )-1 )"
  O1 : Outport
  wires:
  I1/1 -> Fcn/1
  Fcn/1 -> O1/1

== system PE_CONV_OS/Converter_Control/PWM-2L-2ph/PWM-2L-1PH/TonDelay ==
  s1 : Inport  Orientation=down  OutDataType=sfix(16)  OutScaling=2^0
  Int : Integrator  ExternalReset=falling
  Rel1 : Relay  OnSwitchValue=DT  OutDataType=sfix(16)  OutScaling=2^0
  s1d : Outport  InitialOutput=0
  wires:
  Rel1/1 -> s1d/1
  s1/1 -> Int/1, Int/2
  Int/1 -> Rel1/1

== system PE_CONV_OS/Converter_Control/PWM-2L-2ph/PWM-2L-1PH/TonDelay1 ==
  s1 : Inport  Orientation=down  OutDataType=sfix(16)  OutScaling=2^0
  Int : Integrator  ExternalReset=falling
  Rel1 : Relay  OnSwitchValue=DT  OutDataType=sfix(16)  OutScaling=2^0
  s1d : Outport  InitialOutput=0
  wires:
  Rel1/1 -> s1d/1
  s1/1 -> Int/1, Int/2
  Int/1 -> Rel1/1

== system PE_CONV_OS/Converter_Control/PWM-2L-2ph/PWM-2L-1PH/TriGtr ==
  Clock : Clock
  S1 : Subsystem
  Sum : Sum  OutDataType=sfix(16)  OutScaling=2^0
  T : Constant  Value=T  OutDataType=sfix(16)  OutScaling=2^0
  Td : Constant  Value=Td  OutDataType=sfix(16)  OutScaling=2^0
  mod : Math  Operator=mod
  O : Outport  InitialOutput=0
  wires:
  Td/1 -> Sum/2
  Sum/1 -> mod/1
  T/1 -> mod/2
  Clock/1 -> Sum/1
  S1/1(O1) -> O/1
  mod/1 -> S1/1(I1)

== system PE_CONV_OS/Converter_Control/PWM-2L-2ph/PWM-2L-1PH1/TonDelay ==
  s1 : Inport  Orientation=down  OutDataType=sfix(16)  OutScaling=2^0
  Int : Integrator  ExternalReset=falling
  Rel1 : Relay  OnSwitchValue=DT  OutDataType=sfix(16)  OutScaling=2^0
  s1d : Outport  InitialOutput=0
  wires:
  Int/1 -> Rel1/1
  s1/1 -> Int/2, Int/1
  Rel1/1 -> s1d/1

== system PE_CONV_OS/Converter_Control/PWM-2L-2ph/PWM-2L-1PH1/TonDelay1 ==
  s1 : Inport  Orientation=down  OutDataType=sfix(16)  OutScaling=2^0
  Int : Integrator  ExternalReset=falling
  Rel1 : Relay  OnSwitchValue=DT  OutDataType=sfix(16)  OutScaling=2^0
  s1d : Outport  InitialOutput=0
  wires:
  Int/1 -> Rel1/1
  s1/1 -> Int/2, Int/1
  Rel1/1 -> s1d/1

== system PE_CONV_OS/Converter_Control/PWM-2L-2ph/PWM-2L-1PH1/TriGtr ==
  Clock : Clock
  S1 : Subsystem
  Sum : Sum  OutDataType=sfix(16)  OutScaling=2^0
  T : Constant  Value=T  OutDataType=sfix(16)  OutScaling=2^0
  Td : Constant  Value=Td  OutDataType=sfix(16)  OutScaling=2^0
  mod : Math  Operator=mod
  O : Outport  InitialOutput=0
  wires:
  mod/1 -> S1/1(I1)
  S1/1(O1) -> O/1
  Clock/1 -> Sum/1
  T/1 -> mod/2
  Sum/1 -> mod/1
  Td/1 -> Sum/2

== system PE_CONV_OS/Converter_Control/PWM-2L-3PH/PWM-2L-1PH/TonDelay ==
  s1 : Inport  Orientation=down  OutDataType=sfix(16)  OutScaling=2^0
  Int : Integrator  ExternalReset=falling
  Rel1 : Relay  OnSwitchValue=DT  OutDataType=sfix(16)  OutScaling=2^0
  s1d : Outport  InitialOutput=0
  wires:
  Int/1 -> Rel1/1
  s1/1 -> Int/2, Int/1
  Rel1/1 -> s1d/1

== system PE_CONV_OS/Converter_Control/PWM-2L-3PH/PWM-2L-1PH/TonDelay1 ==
  s1 : Inport  Orientation=down  OutDataType=sfix(16)  OutScaling=2^0
  Int : Integrator  ExternalReset=falling
  Rel1 : Relay  OnSwitchValue=DT  OutDataType=sfix(16)  OutScaling=2^0
  s1d : Outport  InitialOutput=0
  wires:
  Int/1 -> Rel1/1
  s1/1 -> Int/2, Int/1
  Rel1/1 -> s1d/1

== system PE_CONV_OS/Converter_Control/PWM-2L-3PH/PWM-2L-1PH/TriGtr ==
  Clock : Clock
  S2 : Subsystem
  Sum : Sum  OutDataType=sfix(16)  OutScaling=2^0
  T : Constant  Value=T  OutDataType=sfix(16)  OutScaling=2^0
  Td : Constant  Value=Td  OutDataType=sfix(16)  OutScaling=2^0
  mod : Math  Operator=mod
  O : Outport  InitialOutput=0
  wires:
  mod/1 -> S2/1(I1)
  S2/1(O1) -> O/1
  Clock/1 -> Sum/1
  T/1 -> mod/2
  Sum/1 -> mod/1
  Td/1 -> Sum/2

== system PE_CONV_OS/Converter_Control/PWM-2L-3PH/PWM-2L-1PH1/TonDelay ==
  s1 : Inport  Orientation=down  OutDataType=sfix(16)  OutScaling=2^0
  Int : Integrator  ExternalReset=falling
  Rel1 : Relay  OnSwitchValue=DT  OutDataType=sfix(16)  OutScaling=2^0
  s1d : Outport  InitialOutput=0
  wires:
  Rel1/1 -> s1d/1
  s1/1 -> Int/1, Int/2
  Int/1 -> Rel1/1

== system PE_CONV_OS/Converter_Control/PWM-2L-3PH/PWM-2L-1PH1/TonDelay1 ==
  s1 : Inport  Orientation=down  OutDataType=sfix(16)  OutScaling=2^0
  Int : Integrator  ExternalReset=falling
  Rel1 : Relay  OnSwitchValue=DT  OutDataType=sfix(16)  OutScaling=2^0
  s1d : Outport  InitialOutput=0
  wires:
  Rel1/1 -> s1d/1
  s1/1 -> Int/1, Int/2
  Int/1 -> Rel1/1

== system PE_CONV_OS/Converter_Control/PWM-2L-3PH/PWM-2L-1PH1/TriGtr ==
  Clock : Clock
  S2 : Subsystem
  Sum : Sum  OutDataType=sfix(16)  OutScaling=2^0
  T : Constant  Value=T  OutDataType=sfix(16)  OutScaling=2^0
  Td : Constant  Value=Td  OutDataType=sfix(16)  OutScaling=2^0
  mod : Math  Operator=mod
  O : Outport  InitialOutput=0
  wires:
  Td/1 -> Sum/2
  Sum/1 -> mod/1
  T/1 -> mod/2
  Clock/1 -> Sum/1
  S2/1(O1) -> O/1
  mod/1 -> S2/1(I1)

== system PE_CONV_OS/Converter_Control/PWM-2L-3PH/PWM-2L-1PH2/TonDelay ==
  s1 : Inport  Orientation=down  OutDataType=sfix(16)  OutScaling=2^0
  Int : Integrator  ExternalReset=falling
  Rel1 : Relay  OnSwitchValue=DT  OutDataType=sfix(16)  OutScaling=2^0
  s1d : Outport  InitialOutput=0
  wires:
  Int/1 -> Rel1/1
  s1/1 -> Int/2, Int/1
  Rel1/1 -> s1d/1

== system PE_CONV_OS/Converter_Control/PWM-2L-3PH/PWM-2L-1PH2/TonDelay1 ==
  s1 : Inport  Orientation=down  OutDataType=sfix(16)  OutScaling=2^0
  Int : Integrator  ExternalReset=falling
  Rel1 : Relay  OnSwitchValue=DT  OutDataType=sfix(16)  OutScaling=2^0
  s1d : Outport  InitialOutput=0
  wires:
  Int/1 -> Rel1/1
  s1/1 -> Int/2, Int/1
  Rel1/1 -> s1d/1

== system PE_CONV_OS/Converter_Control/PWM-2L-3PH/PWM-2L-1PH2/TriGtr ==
  Clock : Clock
  S2 : Subsystem
  Sum : Sum  OutDataType=sfix(16)  OutScaling=2^0
  T : Constant  Value=T  OutDataType=sfix(16)  OutScaling=2^0
  Td : Constant  Value=Td  OutDataType=sfix(16)  OutScaling=2^0
  mod : Math  Operator=mod
  O : Outport  InitialOutput=0
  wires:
  mod/1 -> S2/1(I1)
  S2/1(O1) -> O/1
  Clock/1 -> Sum/1
  T/1 -> mod/2
  Sum/1 -> mod/1
  Td/1 -> Sum/2

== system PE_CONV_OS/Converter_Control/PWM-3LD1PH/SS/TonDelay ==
  s1 : Inport  Orientation=down  OutDataType=sfix(16)  OutScaling=2^0
  Int : Integrator  ExternalReset=falling
  Rel1 : Relay  OnSwitchValue=DT  OutDataType=sfix(16)  OutScaling=2^0
  s1d : Outport  InitialOutput=0
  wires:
  Rel1/1 -> s1d/1
  s1/1 -> Int/1, Int/2
  Int/1 -> Rel1/1

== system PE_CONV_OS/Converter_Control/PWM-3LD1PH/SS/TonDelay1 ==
  s1 : Inport  Orientation=down  OutDataType=sfix(16)  OutScaling=2^0
  Int : Integrator  ExternalReset=falling
  Rel1 : Relay  OnSwitchValue=DT  OutDataType=sfix(16)  OutScaling=2^0
  s1d : Outport  InitialOutput=0
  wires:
  Rel1/1 -> s1d/1
  s1/1 -> Int/1, Int/2
  Int/1 -> Rel1/1

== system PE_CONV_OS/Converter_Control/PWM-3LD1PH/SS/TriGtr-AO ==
  Ampl. : Gain  Gain=A  ParameterDataType=sfix(16)  ParameterScaling=2^0  OutDataType=sfix(16)  OutScaling=2^0
  Offset : Constant  Value=O  OutDataType=sfix(16)  OutScaling=2^0
  Sum : Sum  OutDataType=sfix(16)  OutScaling=2^0
  TriGtr1 : Subsystem  mask(TriGtr){T=T, Td=Td}
      mask prompts: T "Period Time"; Td "Time Delay"
      mask help: Triangular Wave Generator with variable time delay
  Out1 : Outport
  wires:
  Sum/1 -> Out1/1
  Ampl./1 -> Sum/1
  TriGtr1/1(O) -> Ampl./1
  Offset/1 -> Sum/2

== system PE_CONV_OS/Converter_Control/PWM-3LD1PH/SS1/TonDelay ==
  s1 : Inport  Orientation=down  OutDataType=sfix(16)  OutScaling=2^0
  Int : Integrator  ExternalReset=falling
  Rel1 : Relay  OnSwitchValue=DT  OutDataType=sfix(16)  OutScaling=2^0
  s1d : Outport  InitialOutput=0
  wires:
  Rel1/1 -> s1d/1
  s1/1 -> Int/1, Int/2
  Int/1 -> Rel1/1

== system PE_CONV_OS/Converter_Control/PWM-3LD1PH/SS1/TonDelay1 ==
  s1 : Inport  Orientation=down  OutDataType=sfix(16)  OutScaling=2^0
  Int : Integrator  ExternalReset=falling
  Rel1 : Relay  OnSwitchValue=DT  OutDataType=sfix(16)  OutScaling=2^0
  s1d : Outport  InitialOutput=0
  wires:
  Rel1/1 -> s1d/1
  s1/1 -> Int/1, Int/2
  Int/1 -> Rel1/1

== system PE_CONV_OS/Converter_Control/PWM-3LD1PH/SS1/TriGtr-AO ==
  Ampl. : Gain  Gain=A  ParameterDataType=sfix(16)  ParameterScaling=2^0  OutDataType=sfix(16)  OutScaling=2^0
  Offset : Constant  Value=O  OutDataType=sfix(16)  OutScaling=2^0
  Sum : Sum  OutDataType=sfix(16)  OutScaling=2^0
  TriGtr1 : Subsystem  mask(TriGtr){T=T, Td=Td}
      mask prompts: T "Period Time"; Td "Time Delay"
      mask help: Triangular Wave Generator with variable time delay
  Out1 : Outport
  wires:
  Offset/1 -> Sum/2
  TriGtr1/1(O) -> Ampl./1
  Ampl./1 -> Sum/1
  Sum/1 -> Out1/1

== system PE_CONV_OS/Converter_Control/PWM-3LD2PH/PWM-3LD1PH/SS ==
  I1 : Inport  OutDataType=sfix(16)  OutScaling=2^0
  DT : DataTypeConversion
  DT1 : DataTypeConversion
  Relay : Relay  OutDataType=sfix(16)  OutScaling=2^0
  Sum : Sum  Inputs=+-  OutDataType=sfix(16)  OutScaling=2^0
  TonDelay : Subsystem  mask(TonDelay){DT=DT}
      mask prompts: DT "Dead Time"
      mask help: Turn on dead time to protect against short circuit of the converter leg
  TonDelay1 : Subsystem  mask(TonDelay){DT=DT}
      mask prompts: DT "Dead Time"
      mask help: Turn on dead time to protect against short circuit of the converter leg
  TriGtr-AO : Subsystem  mask(TriGtr-AO){A=A, O=O1, T=1/FT, Td=PHT/FT/180}
      mask prompts: A "Amplitude"; O "Offset"; T "Period Time"; Td "Time Delay"
      mask help: Triangular Wave Generator with variable time delay, variable amplitude and offset
  not : Logic  Operator=NOT  Inputs=1
  O1 : Outport  InitialOutput=0
  O2 : Outport  Port=2  InitialOutput=0
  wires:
  DT1/1 -> not/1
  DT/1 -> TonDelay1/1(s1)
  I1/1 -> Sum/1
  TriGtr-AO/1(Out1) -> Sum/2
  Sum/1 -> Relay/1
  not/1 -> DT/1
  TonDelay1/1(s1d) -> O2/1
  Relay/1 -> DT1/1, TonDelay/1(s1)
  TonDelay/1(s1d) -> O1/1

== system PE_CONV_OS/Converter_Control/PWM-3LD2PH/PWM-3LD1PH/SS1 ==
  I1 : Inport  OutDataType=sfix(16)  OutScaling=2^0
  DT : DataTypeConversion
  DT1 : DataTypeConversion
  Relay : Relay  OutDataType=sfix(16)  OutScaling=2^0
  Sum : Sum  Inputs=+-  OutDataType=sfix(16)  OutScaling=2^0
  TonDelay : Subsystem  mask(TonDelay){DT=DT}
      mask prompts: DT "Dead Time"
      mask help: Turn on dead time to protect against short circuit of the converter leg
  TonDelay1 : Subsystem  mask(TonDelay){DT=DT}
      mask prompts: DT "Dead Time"
      mask help: Turn on dead time to protect against short circuit of the converter leg
  TriGtr-AO : Subsystem  mask(TriGtr-AO){A=A, O=O2, T=1/FT, Td=PHT/FT/180}
      mask prompts: A "Amplitude"; O "Offset"; T "Period Time"; Td "Time Delay"
      mask help: Triangular Wave Generator with variable time delay, variable amplitude and offset
  not : Logic  Operator=NOT  Inputs=1
  O1 : Outport  InitialOutput=0
  O2 : Outport  Port=2  InitialOutput=0
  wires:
  DT1/1 -> not/1
  DT/1 -> TonDelay1/1(s1)
  I1/1 -> Sum/1
  TriGtr-AO/1(Out1) -> Sum/2
  Sum/1 -> Relay/1
  not/1 -> DT/1
  TonDelay1/1(s1d) -> O2/1
  Relay/1 -> DT1/1, TonDelay/1(s1)
  TonDelay/1(s1d) -> O1/1

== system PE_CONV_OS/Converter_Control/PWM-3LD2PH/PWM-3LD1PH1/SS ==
  I1 : Inport  OutDataType=sfix(16)  OutScaling=2^0
  DT : DataTypeConversion
  DT1 : DataTypeConversion
  Relay : Relay  OutDataType=sfix(16)  OutScaling=2^0
  Sum : Sum  Inputs=+-  OutDataType=sfix(16)  OutScaling=2^0
  TonDelay : Subsystem  mask(TonDelay){DT=DT}
      mask prompts: DT "Dead Time"
      mask help: Turn on dead time to protect against short circuit of the converter leg
  TonDelay1 : Subsystem  mask(TonDelay){DT=DT}
      mask prompts: DT "Dead Time"
      mask help: Turn on dead time to protect against short circuit of the converter leg
  TriGtr-AO : Subsystem  mask(TriGtr-AO){A=A, O=O1, T=1/FT, Td=PHT/FT/180}
      mask prompts: A "Amplitude"; O "Offset"; T "Period Time"; Td "Time Delay"
      mask help: Triangular Wave Generator with variable time delay, variable amplitude and offset
  not : Logic  Operator=NOT  Inputs=1
  O1 : Outport  InitialOutput=0
  O2 : Outport  Port=2  InitialOutput=0
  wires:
  TonDelay/1(s1d) -> O1/1
  Relay/1 -> TonDelay/1(s1), DT1/1
  TonDelay1/1(s1d) -> O2/1
  not/1 -> DT/1
  Sum/1 -> Relay/1
  TriGtr-AO/1(Out1) -> Sum/2
  I1/1 -> Sum/1
  DT/1 -> TonDelay1/1(s1)
  DT1/1 -> not/1

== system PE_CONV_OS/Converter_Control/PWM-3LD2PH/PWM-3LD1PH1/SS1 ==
  I1 : Inport  OutDataType=sfix(16)  OutScaling=2^0
  DT : DataTypeConversion
  DT1 : DataTypeConversion
  Relay : Relay  OutDataType=sfix(16)  OutScaling=2^0
  Sum : Sum  Inputs=+-  OutDataType=sfix(16)  OutScaling=2^0
  TonDelay : Subsystem  mask(TonDelay){DT=DT}
      mask prompts: DT "Dead Time"
      mask help: Turn on dead time to protect against short circuit of the converter leg
  TonDelay1 : Subsystem  mask(TonDelay){DT=DT}
      mask prompts: DT "Dead Time"
      mask help: Turn on dead time to protect against short circuit of the converter leg
  TriGtr-AO : Subsystem  mask(TriGtr-AO){A=A, O=O2, T=1/FT, Td=PHT/FT/180}
      mask prompts: A "Amplitude"; O "Offset"; T "Period Time"; Td "Time Delay"
      mask help: Triangular Wave Generator with variable time delay, variable amplitude and offset
  not : Logic  Operator=NOT  Inputs=1
  O1 : Outport  InitialOutput=0
  O2 : Outport  Port=2  InitialOutput=0
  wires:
  TonDelay/1(s1d) -> O1/1
  Relay/1 -> TonDelay/1(s1), DT1/1
  TonDelay1/1(s1d) -> O2/1
  not/1 -> DT/1
  Sum/1 -> Relay/1
  TriGtr-AO/1(Out1) -> Sum/2
  I1/1 -> Sum/1
  DT/1 -> TonDelay1/1(s1)
  DT1/1 -> not/1

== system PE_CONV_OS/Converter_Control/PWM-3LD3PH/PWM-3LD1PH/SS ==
  I1 : Inport  OutDataType=sfix(16)  OutScaling=2^0
  DT : DataTypeConversion
  DT1 : DataTypeConversion
  Relay : Relay  OutDataType=sfix(16)  OutScaling=2^0
  Sum : Sum  Inputs=+-  OutDataType=sfix(16)  OutScaling=2^0
  TonDelay : Subsystem  mask(TonDelay){DT=DT}
      mask prompts: DT "Dead Time"
      mask help: Turn on dead time to protect against short circuit of the converter leg
  TonDelay1 : Subsystem  mask(TonDelay){DT=DT}
      mask prompts: DT "Dead Time"
      mask help: Turn on dead time to protect against short circuit of the converter leg
  TriGtr-AO : Subsystem  mask(TriGtr-AO){A=A, O=O1, T=1/FT, Td=PHT/FT/180}
      mask prompts: A "Amplitude"; O "Offset"; T "Period Time"; Td "Time Delay"
      mask help: Triangular Wave Generator with variable time delay, variable amplitude and offset
  not : Logic  Operator=NOT  Inputs=1
  O1 : Outport  InitialOutput=0
  O2 : Outport  Port=2  InitialOutput=0
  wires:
  DT1/1 -> not/1
  DT/1 -> TonDelay1/1(s1)
  I1/1 -> Sum/1
  TriGtr-AO/1(Out1) -> Sum/2
  Sum/1 -> Relay/1
  not/1 -> DT/1
  TonDelay1/1(s1d) -> O2/1
  Relay/1 -> DT1/1, TonDelay/1(s1)
  TonDelay/1(s1d) -> O1/1

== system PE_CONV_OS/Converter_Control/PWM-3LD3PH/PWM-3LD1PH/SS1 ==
  I1 : Inport  OutDataType=sfix(16)  OutScaling=2^0
  DT : DataTypeConversion
  DT1 : DataTypeConversion
  Relay : Relay  OutDataType=sfix(16)  OutScaling=2^0
  Sum : Sum  Inputs=+-  OutDataType=sfix(16)  OutScaling=2^0
  TonDelay : Subsystem  mask(TonDelay){DT=DT}
      mask prompts: DT "Dead Time"
      mask help: Turn on dead time to protect against short circuit of the converter leg
  TonDelay1 : Subsystem  mask(TonDelay){DT=DT}
      mask prompts: DT "Dead Time"
      mask help: Turn on dead time to protect against short circuit of the converter leg
  TriGtr-AO : Subsystem  mask(TriGtr-AO){A=A, O=O2, T=1/FT, Td=PHT/FT/180}
      mask prompts: A "Amplitude"; O "Offset"; T "Period Time"; Td "Time Delay"
      mask help: Triangular Wave Generator with variable time delay, variable amplitude and offset
  not : Logic  Operator=NOT  Inputs=1
  O1 : Outport  InitialOutput=0
  O2 : Outport  Port=2  InitialOutput=0
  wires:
  DT1/1 -> not/1
  DT/1 -> TonDelay1/1(s1)
  I1/1 -> Sum/1
  TriGtr-AO/1(Out1) -> Sum/2
  Sum/1 -> Relay/1
  not/1 -> DT/1
  TonDelay1/1(s1d) -> O2/1
  Relay/1 -> DT1/1, TonDelay/1(s1)
  TonDelay/1(s1d) -> O1/1

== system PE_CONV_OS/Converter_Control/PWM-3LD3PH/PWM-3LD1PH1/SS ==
  I1 : Inport  OutDataType=sfix(16)  OutScaling=2^0
  DT : DataTypeConversion
  DT1 : DataTypeConversion
  Relay : Relay  OutDataType=sfix(16)  OutScaling=2^0
  Sum : Sum  Inputs=+-  OutDataType=sfix(16)  OutScaling=2^0
  TonDelay : Subsystem  mask(TonDelay){DT=DT}
      mask prompts: DT "Dead Time"
      mask help: Turn on dead time to protect against short circuit of the converter leg
  TonDelay1 : Subsystem  mask(TonDelay){DT=DT}
      mask prompts: DT "Dead Time"
      mask help: Turn on dead time to protect against short circuit of the converter leg
  TriGtr-AO : Subsystem  mask(TriGtr-AO){A=A, O=O1, T=1/FT, Td=PHT/FT/180}
      mask prompts: A "Amplitude"; O "Offset"; T "Period Time"; Td "Time Delay"
      mask help: Triangular Wave Generator with variable time delay, variable amplitude and offset
  not : Logic  Operator=NOT  Inputs=1
  O1 : Outport  InitialOutput=0
  O2 : Outport  Port=2  InitialOutput=0
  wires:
  TonDelay/1(s1d) -> O1/1
  Relay/1 -> TonDelay/1(s1), DT1/1
  TonDelay1/1(s1d) -> O2/1
  not/1 -> DT/1
  Sum/1 -> Relay/1
  TriGtr-AO/1(Out1) -> Sum/2
  I1/1 -> Sum/1
  DT/1 -> TonDelay1/1(s1)
  DT1/1 -> not/1

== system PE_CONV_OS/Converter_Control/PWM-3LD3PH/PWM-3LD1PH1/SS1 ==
  I1 : Inport  OutDataType=sfix(16)  OutScaling=2^0
  DT : DataTypeConversion
  DT1 : DataTypeConversion
  Relay : Relay  OutDataType=sfix(16)  OutScaling=2^0
  Sum : Sum  Inputs=+-  OutDataType=sfix(16)  OutScaling=2^0
  TonDelay : Subsystem  mask(TonDelay){DT=DT}
      mask prompts: DT "Dead Time"
      mask help: Turn on dead time to protect against short circuit of the converter leg
  TonDelay1 : Subsystem  mask(TonDelay){DT=DT}
      mask prompts: DT "Dead Time"
      mask help: Turn on dead time to protect against short circuit of the converter leg
  TriGtr-AO : Subsystem  mask(TriGtr-AO){A=A, O=O2, T=1/FT, Td=PHT/FT/180}
      mask prompts: A "Amplitude"; O "Offset"; T "Period Time"; Td "Time Delay"
      mask help: Triangular Wave Generator with variable time delay, variable amplitude and offset
  not : Logic  Operator=NOT  Inputs=1
  O1 : Outport  InitialOutput=0
  O2 : Outport  Port=2  InitialOutput=0
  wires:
  TonDelay/1(s1d) -> O1/1
  Relay/1 -> TonDelay/1(s1), DT1/1
  TonDelay1/1(s1d) -> O2/1
  not/1 -> DT/1
  Sum/1 -> Relay/1
  TriGtr-AO/1(Out1) -> Sum/2
  I1/1 -> Sum/1
  DT/1 -> TonDelay1/1(s1)
  DT1/1 -> not/1
